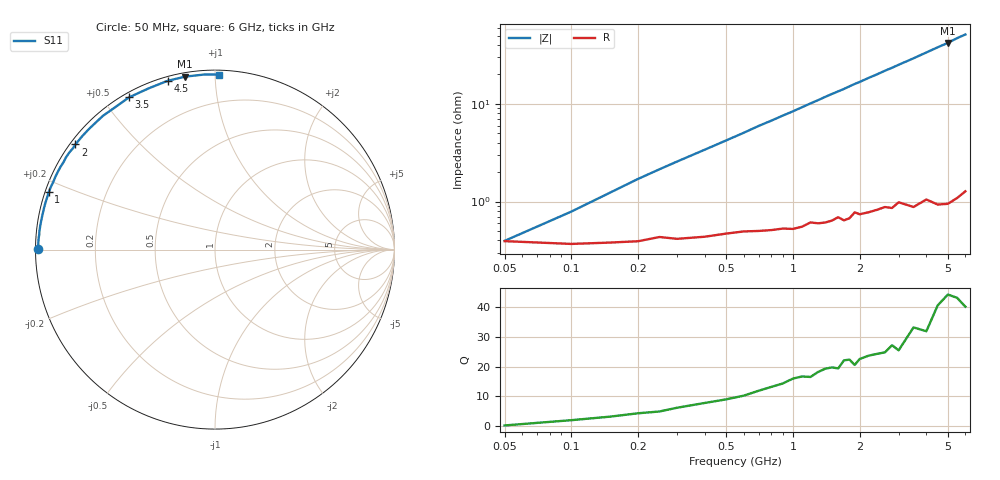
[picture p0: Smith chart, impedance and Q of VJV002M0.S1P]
! Infineon Technologies  Discrete & RF Semiconductors
! BB 914
! Si Tuning Diode in SOT23
! VR =
! S-Parameters:  July  1999
# GHz  S  MA  R  50
!  f  S11
! GHz  MAG  ANG
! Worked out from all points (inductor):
!   34 points, 50 MHz to 6 GHz, reference 50 ohm
!   read as one part to ground: L = 1.32 nH near 150 MHz
!   highest Q = 43.2 at 5 GHz (marker M1), where L = 1.34 nH
!   S11 on the Smith chart (normalised r, x): 50 MHz: 0.01, +0.00; 1 GHz: 0.01, +0.17; 2 GHz: 0.01, +0.33; 3.5 GHz: 0.02, +0.58; 4.5 GHz: 0.02, +0.76; 6 GHz: 0.03, +1.02
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0.05  0.9844 179.9
0.1  0.9854 178.4
0.2  0.9844 176.2
0.25  0.9828 175.2
0.3  0.9836 174.2
0.5  0.9815 170.4
0.7  0.9805 166.5
0.8  0.9801 164.7
1  0.9798 161.0
1.3  0.9774 155.4
1.4  0.9771 153.5
1.5  0.9762 151.7
1.6  0.9745 150.0
1.7  0.9765 148.3
1.8  0.9755 146.4
1.9  0.9722 144.6
2  0.9737 143.0
2.2  0.973 139.5
2.4  0.972 136.3
2.6  0.9709 132.9
2.8  0.9722 129.9
3  0.969 126.7
3.5  0.9741 119.4
4  0.9714 112.3
4.5  0.9766 105.7
5  0.978 99.9
5.5  0.9772 93.6
6  0.9755 88.6
